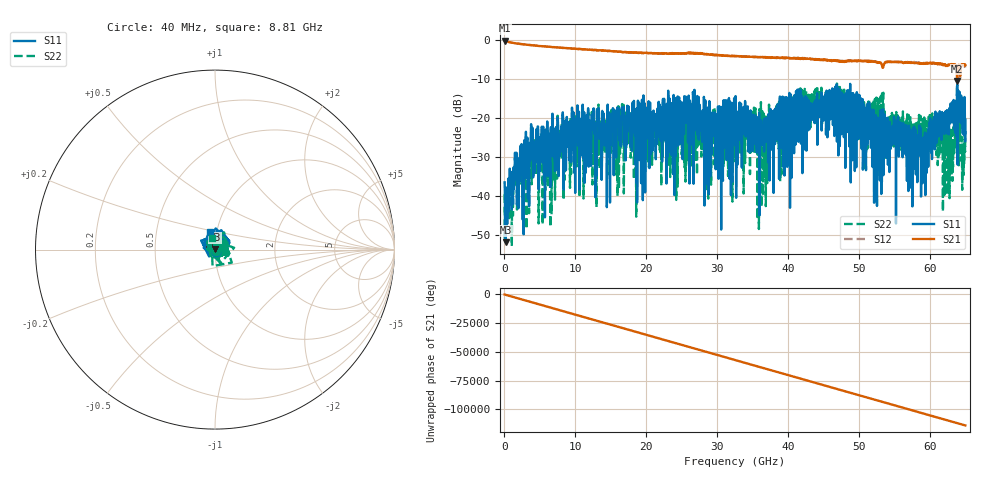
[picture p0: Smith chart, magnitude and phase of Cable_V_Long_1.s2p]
! Created Tue Jul 15 18:11:05 2008
# hz S ma R 50
! 2 Port Network Data from blockName block
! freq  magS11  angS11  magS21  angS21  magS12  angS12  magS22  angS22
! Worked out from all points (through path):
!   1601 points, 40 MHz to 65 GHz, reference 50 ohm
!   highest |S21| = -0.15 dB at 40 MHz (marker M1); lowest = -10.5 dB at 63.82 GHz (marker M2)
!   lowest |S11| = -51.8 dB at 202.4 MHz (marker M3), VSWR 1.01, Z = 49.8 + j0.189 ohm
!   |S11| at or under -10 dB: start of sweep to end of sweep
!   |S22| runs from -52.8 to -11.2 dB; largest |S21 - S12| = 0.049
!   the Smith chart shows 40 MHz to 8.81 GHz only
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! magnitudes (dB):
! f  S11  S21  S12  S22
! 40 MHz  -36.5  -0.2  -0.1  -39.5
! 202.4 MHz  -51.8  -0.3  -0.3  -46.9
! 3.897 GHz  -28.4  -1.4  -1.4  -29.3
! 10.88 GHz  -20.1  -2.4  -2.4  -23.5
! 14.66 GHz  -30.0  -2.8  -2.8  -22.3
! 17.62 GHz  -20.5  -3.2  -3.2  -23.0
! 18.47 GHz  -17.8  -3.3  -3.3  -33.8
! 19.61 GHz  -14.2  -3.4  -3.4  -19.4
! 21.72 GHz  -23.2  -3.4  -3.5  -26.9
! 32.52 GHz  -27.0  -4.1  -4.1  -29.9
! 36.54 GHz  -24.2  -4.4  -4.5  -23.0
! 43.36 GHz  -20.2  -4.9  -4.9  -13.9
! 48.44 GHz  -23.6  -5.4  -5.4  -19.8
! 50.67 GHz  -19.2  -5.5  -5.3  -18.2
! 53.14 GHz  -39.5  -6.1  -6.0  -19.2
! 54.2 GHz  -21.0  -5.6  -5.6  -25.2
! 59.07 GHz  -29.2  -6.1  -6.0  -21.2
! 60.66 GHz  -19.9  -6.1  -6.2  -25.3
! 62.93 GHz  -16.3  -6.4  -6.7  -23.0
! 63.82 GHz  -11.9  -10.5  -10.6  -11.9
! 64.63 GHz  -24.0  -6.3  -6.5  -30.3
! 65 GHz  -20.5  -6.5  -7.1  -23.4
